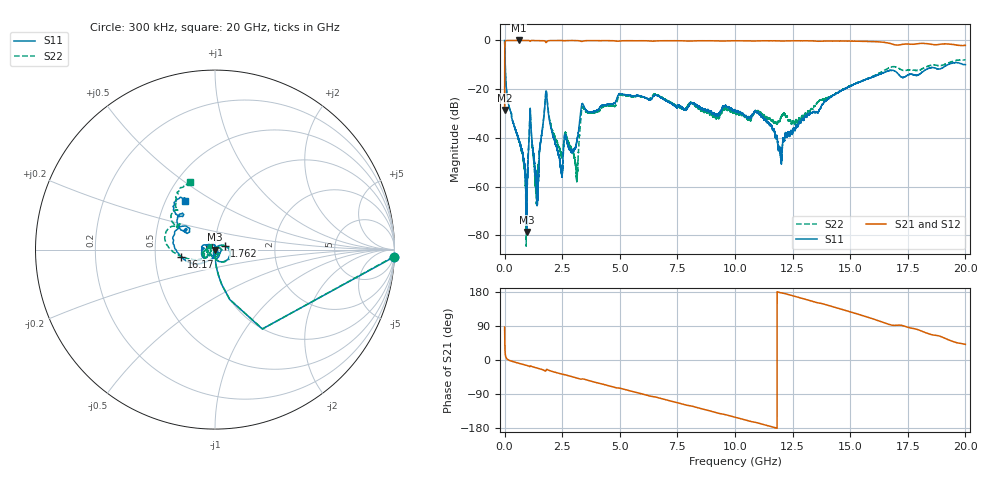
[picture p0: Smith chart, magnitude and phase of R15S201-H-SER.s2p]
!{R15S201}
!Johanson Technology Inc.
!www.johansontechnology.com
!Test Board Conditions:
!Substrate Type  RO4350B
!Substrate Thickness  20 mil
!Substrate Dk  3.66
!TL Type: GCPW
!TL Trace Width  34 mil
!TL Gap  10 mil
!Electrode orientation  Horizontal
!DUT TOPOLOGY	SERIES
!Mounting Pad LxW  26x52 mil
! Created Sat Feb  6 14:20:00 2021
# hz S ma R 50
! 2 Port Network Data from SP1.SP block
! freq  magS11  angS11  magS21  angS21  magS12  angS12  magS22  angS22
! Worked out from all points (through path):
!   20001 points, 300 kHz to 20 GHz, reference 50 ohm
!   highest |S21| = 0.00 dB at 622.3 MHz (marker M1); lowest = -28.5 dB at 300 kHz (marker M2)
!   group delay of S21, straight-line fit = 44.2 ps
!   lowest |S11| = -78.6 dB at 958.3 MHz (marker M3), VSWR 1.00, Z = 50 - j0.01 ohm
!   |S11| at or under -10 dB: 23.95 MHz to 19.23 GHz (19.2 GHz wide, 200 % of centre)
!   |S22| runs from -84.5 to 0.0 dB; largest |S21 - S12| = 0.016
!   S11 on the Smith chart (normalised r, x): 300 kHz: 3, -48; 1.762 GHz: 1.11, +0.05; 16.17 GHz: 0.68, -0.06; 20 GHz: 0.62, +0.37
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300000  0.9976 -2.4  0.03751 87.0  0.03761 87.5  0.9963 -2.3
1.063e8  0.07596 -87.1  0.9969 2.7  0.9965 2.6  0.07648 -87.2
6.223e8  0.009075 -98.7  0.9999 -8.7  0.9977 -8.7  0.008784 -100.3
9.583e8  0.0001171 -121.0  0.9984 -14.3  0.9987 -14.3  0.0009748 85.0
1.0693e9  0.01171 51.7  0.9941 -16.7  0.9942 -16.6  0.01244 55.7
1.1383e9  0.01981 -83.1  0.9898 -16.0  0.9895 -16.0  0.01972 -76.3
1.3133e9  0.002348 -123.9  0.9984 -19.6  0.999 -19.5  0.001631 -76.4
1.4123e9  0.000925 162.2  0.9985 -21.3  0.9985 -21.3  0.001282 34.2
1.7623e9  0.05788 22.2  0.9596 -29.1  0.9595 -29.1  0.06021 21.4
2.4423e9  0.00223 -116.4  0.9958 -36.5  0.9963 -36.5  0.004858 -87.7
2.6813e9  0.009173 -106.9  0.9928 -39.9  0.9934 -39.9  0.01102 -102.2
3.1143e9  0.007387 -52.9  0.993 -47.2  0.9936 -47.2  0.001943 -125.4
3.3343e9  0.04422 -60.9  0.9583 -50.4  0.9577 -50.4  0.03397 -59.3
5.0473e9  0.08042 -155.7  0.98 -75.0  0.9794 -75.0  0.07509 -156.6
6.6673e9  0.07263 161.2  0.9827 -99.5  0.9828 -99.5  0.07427 -166.6
1.00003e10  0.03595 136.6  0.9841 -151.1  0.9842 -151.0  0.03269 124.3
1.10373e10  0.03091 107.7  0.9814 -167.0  0.9812 -167.0  0.03384 125.7
1.19593e10  0.005288 59.6  0.9768 177.8  0.9772 177.8  0.02309 170.8
1.33343e10  0.03294 -97.0  0.9802 155.4  0.9795 155.3  0.03926 -133.7
1.61743e10  0.193 -168.3  0.9398 104.6  0.9376 104.8  0.2026 -170.4
1.66673e10  0.2359 168.3  0.8837 94.1  0.8708 94.3  0.2716 174.0
2e10  0.3181 122.1  0.7918 41.2  0.7854 41.2  0.3993 110.0
